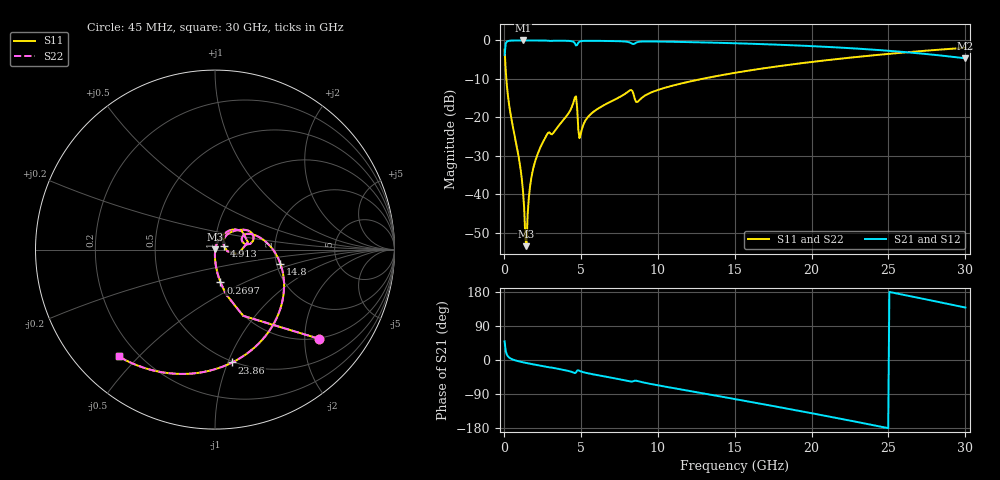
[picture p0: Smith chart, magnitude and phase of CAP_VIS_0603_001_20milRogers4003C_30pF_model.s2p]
! S-parameter model data by Modelithics Inc.  support@modelithics.com  813-866-6335  Tampa FL USA
! S-Parameter data specifications:
! Substrate: 20-mil Rogers 4003C, substrate thickness, H=0.508mm, Dielectric constant, Er=3.75
! PCB Mounting Pad Footprint: Pad width, PadW=0.90mm , Pad length, PadL=1.00mm , Pad gap, PadG (edge-to-edge)=1.00mm , Reference planes=3.0mm apart
! Created Wed Nov 18 13:27:59 2015
# hz S ma R 50
! 2 Port Network Data from SP1.SP block
! freq  magS11  angS11  magS21  angS21  magS12  angS12  magS22  angS22
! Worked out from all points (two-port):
!   401 points, 45 MHz to 30 GHz, reference 50 ohm
!   highest |S21| = -0.01 dB at 1.243 GHz (marker M1); lowest = -4.7 dB at 30 GHz (marker M2)
!   |S21| within 3 dB of the highest: 63.69 MHz to 26.01 GHz (25.95 GHz wide, 199 % of centre)
!   lowest |S11| = -53.4 dB at 1.468 GHz (marker M3), VSWR 1.00, Z = 50.2 + j0.135 ohm
!   |S11| at or under -10 dB: 159.9 MHz to 12.87 GHz (12.71 GHz wide, 195 % of centre)
!   |S22| runs from -53.4 to -1.9 dB; largest |S21 - S12| = 0
!   S11 on the Smith chart (normalised r, x): 45 MHz: 0.99, -2.33; 269.7 MHz: 0.99, -0.38; 4.913 GHz: 1.11, +0.04; 14.8 GHz: 2.10, -0.39; 23.86 GHz: 0.49, -1.04; 30 GHz: 0.13, -0.44
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4.5e7  0.761 -40.7  0.6486 49.3  0.6486 49.3  0.761 -40.7
2.696625e8  0.1858 -80.5  0.9819 9.3  0.9819 9.3  0.1858 -80.5
1.018538e9  0.02603 -91.3  0.9984 -4.0  0.9984 -4.0  0.02603 -91.3
1.2432e9  0.01091 -89.1  0.9985 -6.1  0.9985 -6.1  0.01091 -89.1
1.318088e9  0.006604 -84.8  0.9985 -6.7  0.9985 -6.7  0.006604 -84.8
1.467862e9  0.002131 39.3  0.9984 -8.0  0.9984 -8.0  0.002131 39.3
1.917188e9  0.02222 74.0  0.9979 -11.6  0.9979 -11.6  0.02222 74.0
2.74095e9  0.05707 67.3  0.9935 -18.0  0.9935 -18.0  0.05707 67.3
4.53825e9  0.161 44.5  0.9535 -33.4  0.9535 -33.4  0.161 44.5
4.688025e9  0.1882 12.9  0.8592 -32.9  0.8592 -32.9  0.1882 12.9
4.912688e9  0.05371 20.2  0.9634 -28.6  0.9634 -28.6  0.05371 20.2
5.062462e9  0.06957 46.0  0.9816 -31.0  0.9816 -31.0  0.06957 46.0
5.73645e9  0.1147 50.1  0.9878 -37.3  0.9878 -37.3  0.1147 50.1
8.13285e9  0.2209 26.6  0.9475 -56.2  0.9475 -56.2  0.2209 26.6
8.73195e9  0.1622 23.1  0.9556 -55.9  0.9556 -55.9  0.1622 23.1
1.007992e10  0.2298 21.3  0.9665 -67.3  0.9665 -67.3  0.2298 21.3
1.479784e10  0.373 -12.3  0.9213 -101.5  0.9213 -101.5  0.373 -12.3
1.50225e10  0.3796 -13.9  0.9186 -103.1  0.9186 -103.1  0.3796 -13.9
2.003996e10  0.526 -51.3  0.8424 -140.7  0.8424 -140.7  0.526 -51.3
2.385922e10  0.6359 -81.3  0.7622 -170.7  0.7622 -170.7  0.6359 -81.3
2.505742e10  0.6699 -91.0  0.7324 179.6  0.7324 179.6  0.6699 -91.0
3e10  0.8015 -132.1  0.5849 138.4  0.5849 138.4  0.8015 -132.1
